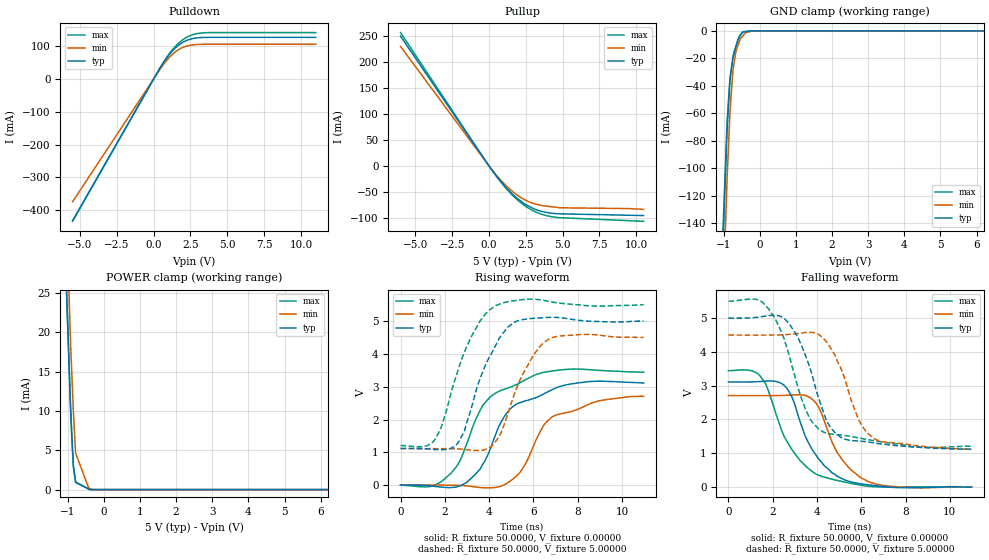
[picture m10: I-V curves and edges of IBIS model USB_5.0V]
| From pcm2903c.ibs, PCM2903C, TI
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[Model] USB_5.0V
Model_type I/O
Vinl  = 0.8V
Vinh  = 2.0V
Vref  = 0.90000V
Rref  = 50.0000ohms
Cref  = 2.00000pF
Vmeas = 2.5000V
C_comp  3.228pF   3.041pF   4.839pF
| variable   typ   min   max
[Voltage Range]   5.00000V  4.50000V  5.50000V
[POWER Clamp Reference]  5.00000V  4.50000V  5.50000V
[Pullup Reference]   5.00000V  4.50000V  5.50000V
[Pulldown Reference]   0.00000V  0.00000V  0.00000V
[GND Clamp Reference]   0.00000V  0.00000V  0.00000V
[Temperature Range]   25   85   -25
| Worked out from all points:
|   slope of the pulldown table from 0 to 0.75 V, typ, clamps not added: 13.6 ohm
|   slope of the pullup table from 0 to 0.75 V, typ, clamps not added: 26.9 ohm
|   GND clamp passes 1 mA (typ) near -0.48 V on its own axis
|   POWER clamp passes 1 mA (typ) near -0.78 V on its own axis
|   rising waveform, R_fixture 50.0000, V_fixture 0.00000: 20-80 % time 1.58ns typ, 1.62ns min, 1.54ns max; typ from 0 V to 3.11 V
|   falling waveform, R_fixture 50.0000, V_fixture 0.00000: 20-80 % time 1.37ns typ, 1.27ns min, 1.53ns max; typ from 3.11 V to 0 V
|   falling waveform, R_fixture 50.0000, V_fixture 5.00000: 20-80 % time 1.21ns typ, 1.2ns min, 1.3ns max; typ from 5 V to 1.12 V
|   rising waveform, R_fixture 50.0000, V_fixture 5.00000: 20-80 % time 1.28ns typ, 1.24ns min, 1.31ns max; typ from 1.12 V to 5 V
[GND Clamp]
-5.5V     -3.403A    -3.781A    -3.24A
-4.5V     -2.679A    -2.982A    -2.55A
-901.2mV  -72.27mA   -107.5mA   -66.23mA
-820.8mV  -36.09mA   -58.69mA   -33.74mA
-739.6mV  -19.22mA   -29.04mA   -19.84mA
-719.5mV  -17.33mA   -25.62mA   -16.41mA
-658.9mV  -11.61mA   -15.3mA    -11.6mA
-603.1mV  -6.34mA    -10.94mA   -7.179mA
-562.2mV  -4.54mA    -7.729mA   -3.928mA
-461.7mV  -920uA     -3.53mA    -703.2uA
-200.4mV  0A         0A         0A
11V       0A         0A         0A
[Pulldown]
-5.5V     -432.1mA   -374.2mA   -434.1mA
279.4mV   21.75mA    18.98mA    21.65mA
658.9mV   49.24mA    43.76mA    50.17mA
1.063V    74.47mA    65.55mA    77.1mA
1.503V    95.64mA    83.8mA     100.4mA
1.902V    109.6mA    94.43mA    117mA
2.221V    117.1mA    99.97mA    126.5mA
2.6V      122.6mA    103.5mA    134.1mA
3.479V    126.6mA    105.6mA    140.9mA
11V       126.8mA    105.7mA    141.4mA
[Pullup]
-6V       250.4mA    230.5mA    257.3mA
39.2mV    -1.888mA   -1.438mA   -1.786mA
620.5mV   -23.75mA   -21.93mA   -24.46mA
1.121V    -40.74mA   -37.25mA   -42.2mA
1.621V    -55.47mA   -50.17mA   -57.51mA
2.081V    -66.41mA   -59.75mA   -69.29mA
2.698V    -78mA      -69.23mA   -81.85mA
3.139V    -83.99mA   -73.53mA   -88.61mA
3.557V    -87.78mA   -76.29mA   -93.35mA
4.301V    -91.58mA   -79.17mA   -98.42mA
4.837V    -92.68mA   -80.99mA   -100.1mA
10.5V     -95.98mA   -84.1mA    -107.1mA
[POWER Clamp]
-6V       688.7mA    805.2mA    684.8mA
-1.281V   58.45mA    74.33mA    58.43mA
-922.5mV  10.59mA    18.82mA    10.86mA
-890.5mV  7.565mA    15.29mA    6.917mA
-841.6mV  2.96mA     9.911mA    2.883mA
-780.6mV  916uA      4.65mA     983.4uA
-420.4mV  70.64uA    213.3uA    75.49uA
-390.3mV  0A         143.1uA    0A
-319.9mV  0A         0A         0A
10.5V     0A         0A         0A
[Rising Waveform]
R_fixture = 50.0000
V_fixture = 0.00000
V_fixture_min = 0.00000
V_fixture_max = 0.00000
0s        0V         0V         0V
1.8ns     -57.41mV   546.8uV    89.3mV
2.52ns    -59.46mV   -4.152mV   557.5mV
3ns       89.55mV    -25.72mV   1.275V
3.72ns    642.5mV    -78.93mV   2.435V
4.44ns    1.795V     -52.7mV    2.856V
5.4ns     2.512V     389.9mV    3.123V
6.36ns    2.742V     1.698V     3.422V
6.84ns    2.907V     2.08V      3.478V
10.98ns   3.11V      2.705V     3.443V
[Falling Waveform]
R_fixture = 50.0000
V_fixture = 0.00000
V_fixture_min = 0.00000
V_fixture_max = 0.00000
0s        3.11V      2.705V     3.443V
1.44ns    3.122V     2.703V     3.279V
1.8ns     3.138V     2.706V     2.86V
2.52ns    3.007V     2.711V     1.489V
2.88ns    2.646V     2.724V     1.095V
3.96ns    937.5mV    2.48V      381.9mV
4.92ns    314.5mV    1.006V     192.3mV
6ns       89.87mV    266.5mV    50.41mV
7.32ns    -6.881mV   20.15mV    -4.144mV
10.98ns   0V         0V         0V
[Falling Waveform]
R_fixture = 50.0000
V_fixture = 5.00000
V_fixture_min = 4.50000
V_fixture_max = 5.50000
0s        5V         4.5V       5.5V
1.56ns    5.048V     4.496V     5.457V
2.16ns    5.08V      4.499V     4.914V
2.64ns    4.909V     4.51V      4.114V
3.48ns    3.888V     4.573V     2.3V
4.32ns    2.157V     4.377V     1.615V
5.04ns    1.483V     3.564V     1.542V
5.88ns    1.356V     1.987V     1.452V
6.36ns    1.327V     1.544V     1.394V
10.98ns   1.122V     1.11V      1.208V
[Rising Waveform]
R_fixture = 50.0000
V_fixture = 5.00000
V_fixture_min = 4.50000
V_fixture_max = 5.50000
0s        1.122V     1.11V      1.208V
1.56ns    1.085V     1.111V     1.392V
2.52ns    1.226V     1.108V     3.338V
2.88ns    1.632V     1.089V     4.046V
3.36ns    2.748V     1.056V     4.728V
4.32ns    4.289V     1.351V     5.481V
4.8ns     4.791V     2.079V     5.585V
5.64ns    5.058V     3.527V     5.662V
6.72ns    5.115V     4.463V     5.598V
10.98ns   5V         4.5V       5.5V
[Ramp]
| variable typ   min   max
dV/dt_r   1.86414/5.28805n  1.62270/5.98045n  2.06123/5.98290n
dV/dt_f   2.32977/5.23878n  2.03342/5.90076n  2.57449/5.03044n
R_load  =  50.0000Ohms
